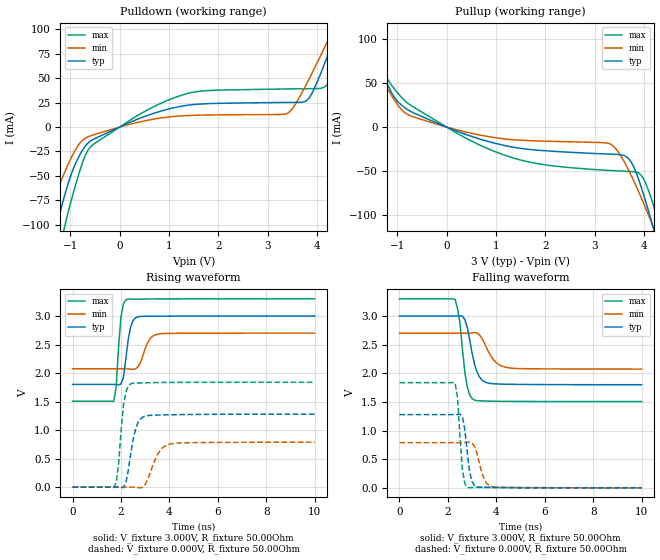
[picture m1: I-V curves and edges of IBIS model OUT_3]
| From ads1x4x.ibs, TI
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|   Output 3.0V Model
[Model]   OUT_3
Model_type   Output
|Signals   nDRDY
| variable   typ   min   max
|C_comp Output average
C_comp   4.426pF   5.188pF   4.249pF
|C_comp Output Low
|C_comp   4.168pF   5.096pF   3.259pF
|C_comp Output High
|C_comp   4.683pF   5.279pF   5.239pF
[Model Spec]
|Timing spec test load voltage corners 0.45*VCC
Vmeas   1.5V   1.35V   1.65V
Vref   1.5V   1.35V   1.65V
|Junction Temperature
[Temperature Range]   40.0   105.0   -40.0
[Voltage range]   5.0V   4.75V   5.25V
[Pullup reference]   3.0V   2.7V   3.3V
[power clamp reference]   3.0V   2.7V   3.3V
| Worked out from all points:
|   slope of the pulldown table from 0 to 0.45 V, typ, clamps not added: 46.1 ohm
|   slope of the pullup table from 0 to 0.45 V, typ, clamps not added: 47.5 ohm
|   falling waveform, V_fixture 3.000V, R_fixture 50.00Ohm: 20-80 % time 369ps typ, 516ps min, 285ps max; typ from 3 V to 1.8 V
|   rising waveform, V_fixture 3.000V, R_fixture 50.00Ohm: 20-80 % time 240ps typ, 344ps min, 176ps max; typ from 1.8 V to 3 V
|   rising waveform, V_fixture 0.000V, R_fixture 50.00Ohm: 20-80 % time 325ps typ, 475ps min, 230ps max; typ from 0 V to 1.28 V
|   falling waveform, V_fixture 0.000V, R_fixture 50.00Ohm: 20-80 % time 216ps typ, 315ps min, 177ps max; typ from 1.28 V to 0 V
[Pulldown]
|   Voltage   I(typ)   I(min)   I(max)
-3V       -489.2mA   -338.7mA   -693.9mA
-1.6V     -168.9mA   -111.3mA   -245.4mA
-1.3V     -105.7mA   -69.5mA    -152.5mA
-1.15V    -76.41mA   -50.51mA   -110.3mA
-650mV    -16.81mA   -10.22mA   -24.24mA
400mV     8.829mA    5.221mA    12.93mA
1.55V     23.28mA    12.1mA     36.2mA
3.4V      25.21mA    14.02mA    39.01mA
3.85V     30.43mA    50.22mA    39.25mA
4.35V     90.84mA    101mA      60.32mA
4.6V      122.4mA    124.1mA    103.4mA
5.95V     234.2mA    208mA      266mA
[Pullup]
|   Voltage   I(typ)   I(min)   I(max)
-3V       210.5mA    183.2mA    247.4mA
-1.95V    135.9mA    115.7mA    162.1mA
-1.6V     97.88mA    83.85mA    115.1mA
-1.2V     48.74mA    43.92mA    55mA
-700mV    16.87mA    12.11mA    23.75mA
1.25V     -21.72mA   -13.81mA   -33.22mA
3.35V     -30.75mA   -20.25mA   -49.29mA
3.75V     -40.26mA   -55.56mA   -50.39mA
3.95V     -68.74mA   -80.47mA   -54.8mA
4.2V      -116.1mA   -114.9mA   -89.62mA
4.3V      -136.6mA   -129.4mA   -112.7mA
5.95V     -512mA     -401.8mA   -635.1mA
[Ramp]
R_load = 50.00Ohm
|   typ   min   max
dV/dt_r   767.516mV/324.646ps 473.345mV/474.679ps   1.103V/229.824ps
dV/dt_f   719.578mV/369.251ps 375.497mV/515.759ps   1.076V/285.154ps
[Falling Waveform]
V_fixture = 3.000V
V_fixture_min = 2.700V
V_fixture_max = 3.300V
R_fixture = 50.00Ohm
|   Time   V(typ)   V(min)   V(max)
0s        3V         2.7V       3.3V
2.3ns     3V         2.7V       3.292V
2.5ns     3.002V     2.7V       2.878V
2.7ns     2.938V     2.7V       2.021V
2.8ns     2.804V     2.7V       1.762V
3.1ns     2.162V     2.712V     1.533V
3.5ns     1.854V     2.537V     1.517V
3.9ns     1.817V     2.229V     1.513V
4.4ns     1.81V      2.104V     1.51V
10ns      1.801V     2.074V     1.507V
[Rising Waveform]
V_fixture = 3.000V
V_fixture_min = 2.700V
V_fixture_max = 3.300V
R_fixture = 50.00Ohm
|   Time   V(typ)   V(min)   V(max)
0s        1.801V     2.074V     1.507V
1.7ns     1.8V       2.074V     1.504V
1.8ns     1.798V     2.074V     1.754V
2ns       1.809V     2.074V     2.985V
2.2ns     2.247V     2.073V     3.282V
2.4ns     2.812V     2.068V     3.298V
2.7ns     2.986V     2.106V     3.295V
3.1ns     2.994V     2.533V     3.297V
3.5ns     2.996V     2.68V      3.298V
10ns      3V         2.7V       3.3V
[Rising Waveform]
V_fixture = 0.000V
V_fixture_min = 0.000V
V_fixture_max = 0.000V
R_fixture = 50.00Ohm
|   Time   V(typ)   V(min)   V(max)
0s        793.8pV    878.1pV    783.1pV
1.7ns     142.2uV    -3.825uV   -7.016mV
1.9ns     -217.4uV   990.3nV    401.1mV
2.1ns     -7.214mV   76.39uV    1.423V
2.4ns     577.1mV    622.9uV    1.812V
2.7ns     1.129V     -8.075mV   1.826V
3ns       1.245V     46.76mV    1.829V
3.5ns     1.264V     565.5mV    1.833V
4ns       1.268V     752.2mV    1.835V
10ns      1.279V     788.9mV    1.838V
[Falling Waveform]
V_fixture = 0.000V
V_fixture_min = 0.000V
V_fixture_max = 0.000V
R_fixture = 50.00Ohm
|   Time   V(typ)   V(min)   V(max)
0s        1.279V     788.9mV    1.838V
2.3ns     1.28V      788.7mV    1.834V
2.4ns     1.282V     788.8mV    1.565V
2.6ns     1.252V     789.9mV    315.3mV
2.8ns     614.8mV    795.5mV    9.752mV
2.9ns     279.3mV    797.1mV    2.401mV
3.1ns     36.64mV    724.7mV    8.427mV
3.5ns     10.17mV    149.6mV    6.538mV
3.8ns     9.03mV     23.93mV    4.597mV
10ns      793.8pV    878.1pV    783.1pV
